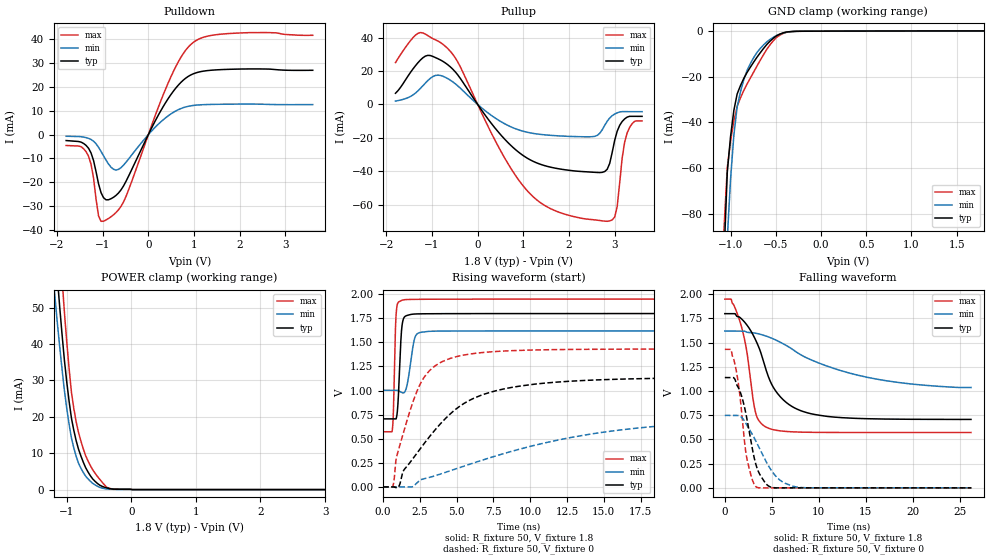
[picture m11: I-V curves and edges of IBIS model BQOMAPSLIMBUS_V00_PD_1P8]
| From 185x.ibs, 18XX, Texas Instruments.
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|   Model Cell BQOMAPSLIMBUS_V00_PD_1P8
|BQOMAPSLIMBUS_V00_PD_1P8
[Model]   BQOMAPSLIMBUS_V00_PD_1P8
Model_type   I/O
Polarity   Non-Inverting
Enable   Active-Low
Vinl =  0.63
Vinh =  1.17
Cref =  15pF
Rref =  100.0000M
Vref =  0V
Vmeas =  0.9
C_comp   1.636035p   1.481314p   1.795483p
[Model Spec]
Vinl   0.63   0.567   0.6825
Vinh   1.17   1.053   1.2675
[Temperature Range]   25   125   -40
[Voltage Range]   1.8   1.62   1.95
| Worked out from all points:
|   slope of the pulldown table from 0 to 0.27 V, typ, clamps not added: 27.2 ohm
|   slope of the pullup table from 0 to 0.27 V, typ, clamps not added: 26.2 ohm
|   GND clamp passes 1 mA (typ) near -0.44 V on its own axis
|   POWER clamp passes 1 mA (typ) near -0.46 V on its own axis
|   rising waveform, R_fixture 50, V_fixture 1.8: 20-80 % time 199ps typ, 360ps min, 134ps max; typ from 0.706 V to 1.8 V
|   rising waveform, R_fixture 50, V_fixture 0: 20-80 % time 4.31ns typ, 10.1ns min, 1.94ns max; typ from 0 V to 1.14 V
|   falling waveform, R_fixture 50, V_fixture 1.8: 20-80 % time 3.05ns typ, 8.7ns min, 1.37ns max; typ from 1.8 V to 0.706 V
|   falling waveform, R_fixture 50, V_fixture 0: 20-80 % time 1.45ns typ, 2.53ns min, 1.05ns max; typ from 1.14 V to 0 V
| Nom Voltages:
|   BIASFET=1.8, VBBNW=1.1, VDD=1.1, VDDS=1.8, VDDU=1.05, VSS=0, VSSS=0
| Min Voltages:
|   BIASFET=1.62, VBBNW=0.99, VDD=0.99, VDDS=1.62, VDDU=0.95, VSS=0,
|   VSSS=0
| Max Voltages:
|   BIASFET=1.95, VBBNW=1.21, VDD=1.21, VDDS=1.95, VDDU=1.16, VSS=0,
|   VSSS=0
[POWER_clamp]
|   voltage   I(typ)   I(min)   I(max)
-1.8V     243.4mA    191.6mA    307.8mA
-1.182V   67.14mA    52.87mA    87.8mA
-1.109V   50.26mA    39.3mA     67.51mA
-1.073V   42.68mA    33.12mA    58mA
-1.036V   35.59mA    27.28mA    48.82mA
-963.6mV  24.31mA    18.01mA    33.31mA
-927.3mV  19.65mA    14.2mA     26.77mA
-854.5mV  13.48mA    9.176mA    18.67mA
-709.1mV  6.095mA    3.747mA    9.4mA
-527.3mV  1.73mA     943.2uA    3.675mA
-272.7mV  118.9uA    74.64uA    178uA
3.6V      0A         0A         0A
[Pulldown]
|   voltage   I(typ)   I(min)   I(max)
-1.8V     -2.487mA   -681.8uA   -4.562mA
-1.473V   -3.152mA   -884.6uA   -5.067mA
-1.309V   -5.739mA   -1.559mA   -9.111mA
-1.2V     -10.86mA   -2.75mA    -18.26mA
-1.091V   -20.62mA   -5.298mA   -34.07mA
-981.8mV  -26.44mA   -8.861mA   -36.31mA
-654.5mV  -24.49mA   -14.59mA   -31.53mA
-436.4mV  -17.53mA   -10.31mA   -23.34mA
381.8mV   13.54mA    7.116mA    19.31mA
927.3mV   25mA       12.07mA    37.76mA
1.691V    27.34mA    12.75mA    42.29mA
3.6V      26.98mA    12.59mA    41.65mA
[Pullup]
|   voltage   I(typ)   I(min)   I(max)
-1.8V     6.703mA    2.011mA    25.06mA
-1.309V   24.97mA    8.116mA    42.58mA
-709.1mV  24.88mA    16.26mA    34.85mA
927.3mV   -29.26mA   -15.5mA    -46.38mA
1.418V    -36.26mA   -18.07mA   -59.68mA
2.127V    -39.86mA   -19.24mA   -67.34mA
2.782V    -40.19mA   -12.5mA    -69.92mA
3V        -21.5mA    -5.748mA   -67.44mA
3.055V    -16.07mA   -5.025mA   -61.28mA
3.164V    -10.24mA   -4.312mA   -32.15mA
3.273V    -7.595mA   -4.315mA   -17.08mA
3.6V      -7.13mA    -4.323mA   -9.859mA
[GND_clamp]
|   voltage   I(typ)   I(min)   I(max)
-1.8V     -5.104A    -4.871A    -5.301A
-1.073V   -99.01mA   -143.7mA   -86.51mA
-1.036V   -61.78mA   -90.71mA   -59.81mA
-1V       -46.11mA   -64.73mA   -48.24mA
-963.6mV  -34.7mA    -45.54mA   -39.29mA
-927.3mV  -27.54mA   -33.17mA   -32.95mA
-890.9mV  -23.9mA    -26.66mA   -29.29mA
-818.2mV  -18.14mA   -17.24mA   -23.2mA
-745.5mV  -13.61mA   -11.65mA   -17.98mA
-527.3mV  -3.104mA   -2.701mA   -4.21mA
-272.7mV  -55.4uA    -76.65uA   -80.17uA
1.8V      92.49uA    51.14uA    157.6uA
[Ramp]
| variable   typ   min   max
dV/dt_f 0.65748115/3.0608237n 0.37065581/9.87254n   0.82818558/1.3821932n
dV/dt_r 0.68927974/4.3650001n 0.45362211/12.396313n 0.86514692/1.9395091n
R_load = 50
[Rising Waveform]
R_fixture = 50
V_fixture = 1.8
V_fixture_min = 1.62
V_fixture_max = 1.95
|   time   V(typ)   V(min)   V(max)
0s        705.6mV    1.003V     572.1mV
630.8ps   705.6mV    1.003V     601.6mV
704.2ps   705.6mV    1.003V     822.4mV
832.2ps   705.6mV    1.003V     1.626V
912ps     724.5mV    1.003V     1.846V
1.296ns   1.688V     976.9mV    1.937V
1.615ns   1.778V     1.049V     1.944V
2.145ns   1.794V     1.543V     1.946V
2.565ns   1.796V     1.604V     1.946V
26.2ns    1.798V     1.619V     1.948V
[Rising Waveform]
R_fixture = 50
V_fixture = 0
V_fixture_min = 0
V_fixture_max = 0
|   time   V(typ)   V(min)   V(max)
0s        0V         0V         0V
654ps     0V         0V         3.053mV
944.5ps   -9.65mV    0V         330mV
1.392ns   170.6mV    0V         570mV
2.548ns   401.8mV    73.5mV     1.076V
4.494ns   747.7mV    164mV      1.329V
6.645ns   949.8mV    273.1mV    1.392V
10.23ns   1.065V     428.9mV    1.42V
17.11ns   1.122V     607.5mV    1.429V
26.25ns   1.135V     685mV      1.43V
[Falling Waveform]
R_fixture = 50
V_fixture = 1.8
V_fixture_min = 1.62
V_fixture_max = 1.95
|   time   V(typ)   V(min)   V(max)
0s        1.798V     1.618V     1.948V
674.4ps   1.798V     1.618V     1.948V
1.587ns   1.76V      1.618V     1.724V
2.316ns   1.685V     1.608V     1.424V
3.261ns   1.529V     1.597V     781.5mV
4.351ns   1.229V     1.568V     628.8mV
6.024ns   927.4mV    1.497V     586.6mV
8.976ns   769.5mV    1.33V      573.4mV
16.27ns   711.2mV    1.12V      571.3mV
26.2ns    706.2mV    1.036V     571.2mV
[Falling Waveform]
R_fixture = 50
V_fixture = 0
V_fixture_min = 0
V_fixture_max = 0
|   time   V(typ)   V(min)   V(max)
0s        1.138V     747.9mV    1.429V
648.3ps   1.138V     747.9mV    1.429V
1.056ns   1.123V     747.9mV    1.284V
1.539ns   1.015V     747.9mV    1.007V
2.303ns   736.4mV    654mV      325mV
2.87ns    433mV      560.9mV    99.91mV
3.367ns   221.7mV    470.4mV    7.572mV
4.752ns   13.24mV    210mV      0V
7.463ns   0V         11.83mV    0V
26.25ns   0V         0V         0V
